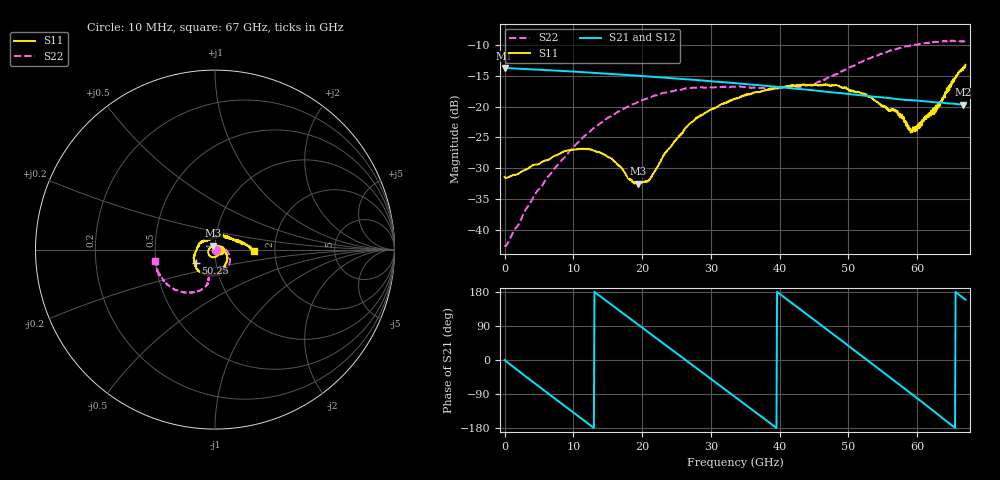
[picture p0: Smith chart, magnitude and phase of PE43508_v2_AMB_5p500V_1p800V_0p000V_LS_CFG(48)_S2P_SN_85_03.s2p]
!Keysight Technologies,N5227A,US51270237,A.10.43.00
!Date: Wednesday, August 22, 2018 17:11:35
!Correction: S11(Full 2 Port(1,3))
!S31(Full 2 Port(1,3))
!S13(Full 2 Port(1,3))
!S33(Full 2 Port(1,3))
!S2P File: Measurements: S11, S31, S13, S33:
# Hz S  dB  R 50
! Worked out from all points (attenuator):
!   801 points, 10 MHz to 67 GHz, reference 50 ohm
!   highest |S21| = -13.71 dB at 10 MHz (marker M1); lowest = -19.7 dB at 66.67 GHz (marker M2)
!   lowest |S11| = -32.5 dB at 19.35 GHz (marker M3), VSWR 1.05, Z = 49.1 + j2.16 ohm
!   |S11| at or under -10 dB: start of sweep to end of sweep
!   |S22| runs from -42.7 to -9.3 dB; largest |S21 - S12| = 0.001
!   S11 on the Smith chart (normalised r, x): 10 MHz: 1.06, -0.00; 50.25 GHz: 0.80, -0.12; 67 GHz: 1.56, -0.03
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1e7  -31.43 -1.3  -13.71 -0.2  -13.71 -0.2  -42.54 -2.1
2.522125e9  -30.54 -32.4  -13.87 -35.7  -13.88 -35.7  -38.06 27.6
5.787888e9  -28.83 -67.0  -14.05 -80.8  -14.06 -80.8  -32.22 29.4
8.300012e9  -27.47 -93.4  -14.21 -115.3  -14.21 -115.3  -28.72 20.7
1.123082e10  -26.84 -121.3  -14.40 -155.4  -14.40 -155.3  -25.23 4.0
1.483154e10  -28.06 -160.7  -14.65 155.6  -14.65 155.6  -21.98 -16.4
1.935336e10  -32.53 111.6  -14.99 94.2  -14.99 94.3  -19.26 -41.3
2.102811e10  -31.83 64.3  -15.13 71.5  -15.12 71.6  -18.59 -49.9
2.236791e10  -29.54 31.0  -15.23 53.4  -15.23 53.4  -18.07 -56.6
2.6806e10  -22.91 -24.3  -15.59 -6.7  -15.59 -6.6  -17.02 -75.9
3.040671e10  -20.35 -49.6  -15.92 -55.4  -15.92 -55.3  -16.89 -88.6
3.3505e10  -18.73 -68.0  -16.20 -97.4  -16.20 -97.3  -16.77 -96.9
3.911541e10  -17.14 -93.5  -16.74 -173.5  -16.74 -173.3  -17.16 -103.4
4.472582e10  -16.52 -118.8  -17.33 109.9  -17.32 109.9  -16.41 -102.3
5.02525e10  -17.55 -145.0  -17.99 33.9  -17.99 33.9  -13.59 -103.9
5.586291e10  -20.72 167.1  -18.61 -43.7  -18.60 -44.0  -10.98 -121.6
5.703524e10  -20.95 157.5  -18.77 -60.0  -18.77 -60.2  -10.59 -126.2
5.89612e10  -23.53 122.1  -18.96 -86.5  -18.96 -86.6  -10.09 -133.7
6.004979e10  -22.99 94.7  -19.03 -101.8  -19.04 -102.1  -9.95 -138.3
6.29806e10  -19.46 42.5  -19.30 -143.2  -19.32 -143.5  -9.51 -150.9
6.666505e10  -14.07 0.8  -19.71 163.9  -19.77 164.0  -9.37 -166.7
6.7e10  -13.20 -2.6  -19.69 159.1  -19.77 159.1  -9.37 -168.8
